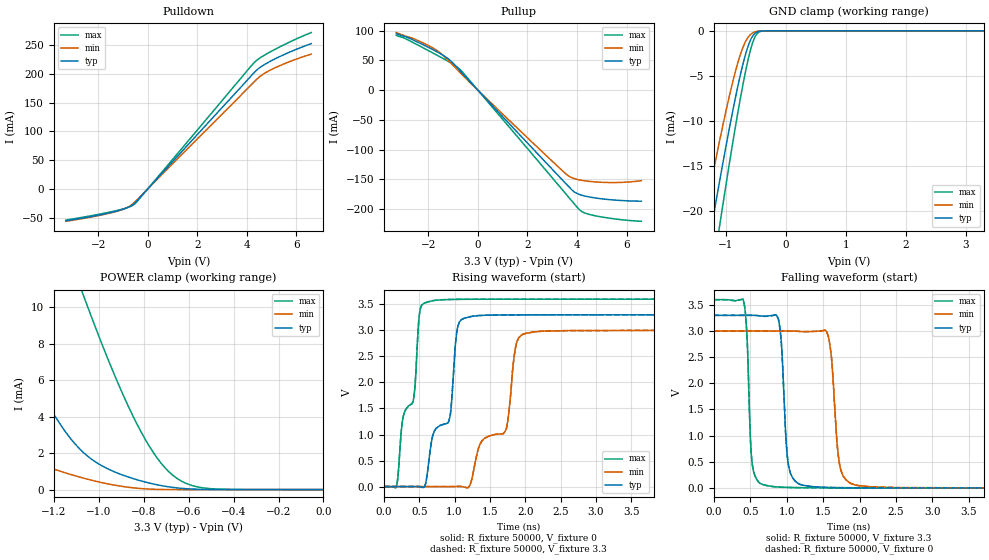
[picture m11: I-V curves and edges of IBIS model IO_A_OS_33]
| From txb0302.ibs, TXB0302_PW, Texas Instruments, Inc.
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[Model]   IO_A_OS_33
Model_type  3-state
Enable   Active-High
Vref =   0
Rref =   50000
Cref =   15p
Vmeas =   1.65
| variable   typ   min   max
C_comp   3.23pF   2.99pF   3.46pF
| C_pullup   0.79pF   0.59pF   1.01pF
| C_pulldown   0.69pF   0.56pF   0.81pF
| C_tri-state   3.23pF   2.99pF   3.46pF
[Temperature Range]   40   100   -40
| Ambient temperature   25   85   -40
[Voltage range]   3.3   3   3.6
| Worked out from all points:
|   slope of the pulldown table from 0 to 0.495 V, typ, clamps not added: 21.1 ohm
|   slope of the pullup table from 0 to 0.495 V, typ, clamps not added: 22.5 ohm
|   GND clamp passes 1 mA (typ) near -0.59 V on its own axis
|   POWER clamp passes 1 mA (typ) near -0.93 V on its own axis
|   rising waveform, R_fixture 50000, V_fixture 0: 20-80 % time 355ps typ, 521ps min, 252ps max; typ from 0 V to 3.3 V
|   falling waveform, R_fixture 50000, V_fixture 3.3: 20-80 % time 72.5ps typ, 90.3ps min, 54.4ps max; typ from 3.3 V to 0.001 V
|   rising waveform, R_fixture 50000, V_fixture 3.3: 20-80 % time 355ps typ, 521ps min, 252ps max; typ from 0.001 V to 3.3 V
|   falling waveform, R_fixture 50000, V_fixture 0: 20-80 % time 72.5ps typ, 90.3ps min, 54.4ps max; typ from 3.3 V to 0 V
[GND Clamp]
| IO_A_33
|   Voltage   I(typ)   I(min)   I(max)
-3.3V     -107.8mA   -94.82mA   -123.5mA
-1.4V     -27.92mA   -22.08mA   -34.6mA
-1.355V   -26.16mA   -20.51mA   -32.58mA
-1.24V    -21.7mA    -16.57mA   -27.47mA
-1.105V   -16.6mA    -12.13mA   -21.56mA
-930mV    -10.32mA   -6.816mA   -14.13mA
-780mV    -5.448mA   -3.031mA   -8.201mA
-650mV    -2.065mA   -895.1uA   -3.734mA
-540mV    -437.9uA   -178.1uA   -1.021mA
-465mV    -87.77uA   -39.15uA   -208.4uA
-365mV    -6.098uA   -3.222uA   -9.086uA
3.3V      878.5pA    29.7nA     71.4pA
[POWER Clamp]
| IO_A_33
|   Voltage   I(typ)   I(min)   I(max)
-3.3V     75.76mA    55.16mA    102.1mA
-1.87V    23.53mA    10.79mA    41.25mA
-1.62V    15.48mA    5.161mA    31.23mA
-1.465V   10.85mA    2.838mA    25.17mA
-1.225V   4.661mA    1.234mA    16.15mA
-1.065V   1.999mA    620.1uA    10.55mA
-935mV    1mA        257uA      6.436mA
-830mV    541.2uA    77.16uA    3.598mA
-740mV    263.8uA    13.45uA    1.73mA
-670mV    119.9uA    2.07uA     782.6uA
-510mV    6.607uA    44.4nA     59.35uA
0V        0A         0A         0A
[Pulldown]
| IO_A_33
|   Voltage   I(typ)   I(min)   I(max)
-3.3V     -55.56mA   -56.47mA   -54.3mA
-2.115V   -46.75mA   -47.57mA   -45.39mA
-1.295V   -39.01mA   -39.55mA   -38.14mA
-835mV    -32.8mA    -32.59mA   -32.87mA
-550mV    -25.56mA   -23.89mA   -26.97mA
-400mV    -18.94mA   -17.51mA   -20.42mA
4.315V    203mA      187.1mA    220.3mA
4.635V    214.1mA    198.7mA    230.6mA
5.08V     224.9mA    209.4mA    241.4mA
5.805V    239.2mA    222.6mA    257mA
6.6V      252.7mA    234.3mA    271.9mA
[Pullup]
| IO_A_33
|   Voltage   I(typ)   I(min)   I(max)
-3.3V     95.24mA    96.92mA    92.38mA
-2.54V    82.96mA    85.65mA    78.42mA
-1.72V    66.06mA    68.5mA     60.38mA
-1.17V    51.86mA    48.76mA    47.82mA
-730mV    32.97mA    29.97mA    35.13mA
2.06V     -91.37mA   -82.32mA   -100.9mA
3.69V     -163mA     -144.8mA   -181.1mA
3.895V    -171mA     -148.6mA   -191.2mA
4.11V     -175.4mA   -150.8mA   -201.3mA
4.39V     -178.5mA   -152.7mA   -207.4mA
5.52V     -184.6mA   -155.2mA   -216.3mA
6.6V      -186.5mA   -152mA     -220.3mA
[Ramp]
| IO_A_33
| variable   typ   min   max
dV/dt_r   1.99/3.57E-10   1.81/5.26E-10   2.17/2.53E-10
dV/dt_f   1.99/7.53E-11   1.81/9.38E-11   2.17/5.58E-11
R_load = 50000
[Rising Waveform]
| IO_A_33
R_fixture =   50000
C_fixture =   0
L_fixture =   0
V_fixture =   0
V_fixture_min = 0
V_fixture_max = 0
|   Time   V(typ)   V(min)   V(max)
0s        2.652nV    9.613nV    576.2pV
181ps     -10.96uV   -10.52nV   27.46mV
421ps     185.9uV    584.1nV    1.697V
517ps     -7.262mV   -4.129uV   3.422V
797ps     1.176V     48.04uV    3.585V
933ps     1.333V     -149uV     3.593V
1.093ns   3.202V     2.194mV    3.596V
1.909ns   3.297V     2.859V     3.598V
2.237ns   3.298V     2.984V     3.598V
37.64ns   3.299V     2.998V     3.599V
[Falling Waveform]
| IO_A_33
R_fixture =   50000
C_fixture =   0
L_fixture =   0
V_fixture =   3.3
V_fixture_min = 3
V_fixture_max = 3.6
|   Time   V(typ)   V(min)   V(max)
0s        3.3V       3V         3.6V
397ps     3.3V       3V         3.61V
533ps     3.3V       3V         381.7mV
885ps     3.22V      3V         16.23mV
1.037ns   340.2mV    3V         7.54mV
1.421ns   16.71mV    2.996V     2.523mV
1.581ns   7.748mV    2.825V     2.051mV
1.757ns   4.136mV    279.3mV    1.798mV
2.165ns   2.023mV    18.47mV    1.583mV
37.64ns   1.393mV    1.375mV    1.408mV
[Rising Waveform]
| IO_A_33
R_fixture =   50000
C_fixture =   0
L_fixture =   0
V_fixture =   3.3
V_fixture_min = 3
V_fixture_max = 3.6
|   Time   V(typ)   V(min)   V(max)
0s        1.391mV    1.369mV    1.407mV
181ps     1.381mV    1.369mV    28.87mV
421ps     1.577mV    1.369mV    1.699V
517ps     -5.87mV    1.365mV    3.424V
797ps     1.177V     1.417mV    3.587V
933ps     1.334V     1.22mV     3.594V
1.093ns   3.203V     3.563mV    3.597V
1.909ns   3.299V     2.86V      3.6V
2.237ns   3.299V     2.985V     3.6V
37.64ns   3.3V       3V         3.6V
[Falling Waveform]
| IO_A_33
R_fixture =   50000
C_fixture =   0
L_fixture =   0
V_fixture =   0
V_fixture_min = 0
V_fixture_max = 0
|   Time   V(typ)   V(min)   V(max)
0s        3.299V     2.998V     3.599V
397ps     3.299V     2.998V     3.608V
533ps     3.298V     2.998V     380.2mV
885ps     3.219V     2.998V     14.82mV
1.037ns   338.7mV    2.998V     6.132mV
1.421ns   15.32mV    2.995V     1.116mV
1.581ns   6.357mV    2.824V     644.3uV
1.757ns   2.745mV    277.8mV    390.4uV
2.165ns   632uV      17.1mV     175.6uV
37.64ns   1.77uV     6.825uV    531.6nV
